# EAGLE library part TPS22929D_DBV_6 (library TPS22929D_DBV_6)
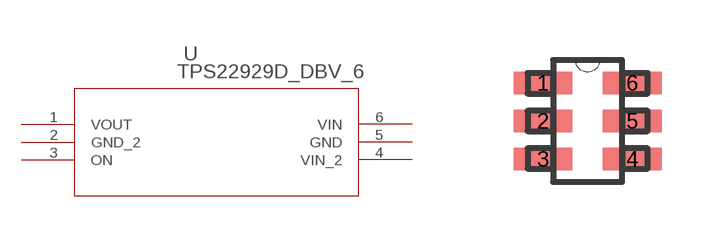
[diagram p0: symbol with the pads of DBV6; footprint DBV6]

Designator prefix U

## TPS22929D_DBV_6 (DATASHEETURL: http://www.ti.com/lit/gpn/TPS22929D; DESCRIPTION: Low Input Voltage, 1.8A Single Channel Load Switch with Controlled Turn-On; FAMILY_NAME: NON CURRENT LIMITED LOAD SWITCH; GENERIC_PART_NUMBER: TPS22929D; INDUSTRY_STD_PKG_TYPE: SOT-23; MANUFACTURER: Texas Instruments; MANUFACTURER_PART_NUMBER: tps22929d_dbv_6; PACKAGE_DESIGNATOR: DBV; PIN_COUNT: 6; VENDOR: Texas Instruments)  [DBV6]
1  VOUT  out
2  GND_2  pwr
3  ON  in
4  VIN_2  in
5  GND  pwr
6  VIN  in

## Footprint DBV6 (pad centres in mm)
smd 1.473 x 0.559: 1 -1.118,0.95; 2 -1.118,0; 3 -1.118,-0.95; 4 1.118,-0.95; 5 1.118,0; 6 1.118,0.95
